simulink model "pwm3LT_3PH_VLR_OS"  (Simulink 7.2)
settings: Solver=ode3  SolverMode=SingleTasking  StartTime=0.0  StopTime=0.1  FixedStep=10e-6  MaxStep=1e-4  RelTol=1e-3

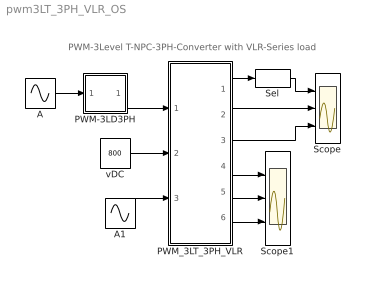
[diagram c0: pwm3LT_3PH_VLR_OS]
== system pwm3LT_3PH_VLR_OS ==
  note: PWM-3Level T-NPC-3PH-Converter with VLR-Series load
  A : Sin  Amplitude=.8  Frequency=2*pi*50  Phase="[0  -2*pi/3  -4*pi/3 ]"  SampleTime=0
  A1 : Sin  Amplitude=0  Frequency=2*pi*50  Phase="[0  -2*pi/3  -4*pi/3 ]"  SampleTime=0
  PWM-3LD3PH : Subsystem  mask(PWM-3LD3PH){FT=900, PHT=0, A=0.5, O1=0.5, O2=-0.5, DT=1e-6}
      mask prompts: FT "Frequency of Trian Sig."; PHT "Phase Angle of Trian. Sig."; A "Amplitude of Trian. Sig."; O1 "Offset of 1st Trian"; O2 "Offset of 2nd Trian."; DT "Dead Time"
      mask help: Pulse Width Modulation for 3 Phase 3 Level Neutral point clamped Converter
  PWM_3LT_3PH_VLR : Subsystem  mask(pwm_3LT_3PH_VLR_OS){RL=1, LL=1e-3}
      mask prompts: RL "Load Resistance"; LL "Load Inductance"
      mask help: Open Source 3-Level T-NPC PWM_3PH Converter with VLR load Input Vector u: u{0:11}= gating Signals u[12]/2= VDC1, VDC2 u{13:15}= EA,EB,EC Output Vector y: y{0:2}= Va,Vb,Vc, Output AC Voltages to middle point y{3:5}= Ia,Ib,Ic, Output AC Currents y[6]= Vab.V, Output Voltage y{7:9} = T1.I,D1.I,T1.V y{10:12}= T2.I,D2.I,T2.V y[13]= D5.I y[14]= D5.V y[15]= IDC1, Input DC Current y[16]= IDC2, Input DC Current Parameter Vector p: p[0]=RL p[1]=LL You can pause the simulation during running, change the Parameters you want and continue the Simulation
  Scope : Scope  NumInputPorts=3
  Scope1 : Scope  NumInputPorts=3
  Sel : Selector  InputPortWidth=3  IndexOptions=Index vector (dialog)  Indices=[1 ]  OutputSizes=1
  vDC : Constant  Value=800  OutDataType=sfix(16)  OutScaling=2^0
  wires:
  A/1 -> PWM-3LD3PH/1(In1)
  A1/1 -> PWM_3LT_3PH_VLR/3(E_ABC)
  vDC/1 -> PWM_3LT_3PH_VLR/2(vDC)
  PWM-3LD3PH/1(Out1) -> PWM_3LT_3PH_VLR/1(Sw)
  PWM_3LT_3PH_VLR/4("iT1, iD1,vT1") -> Scope1/1
  PWM_3LT_3PH_VLR/5("iT2, iD2,vT2") -> Scope1/2
  PWM_3LT_3PH_VLR/6(iDC1,iDC2) -> Scope1/3
  PWM_3LT_3PH_VLR/1(vABC) -> Sel/1
  PWM_3LT_3PH_VLR/2(iABC) -> Scope/2
  PWM_3LT_3PH_VLR/3(vAB) -> Scope/3
  Sel/1 -> Scope/1

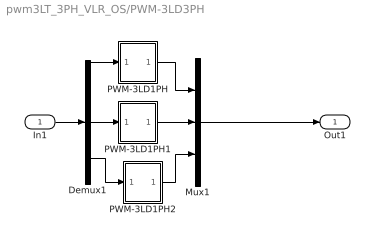
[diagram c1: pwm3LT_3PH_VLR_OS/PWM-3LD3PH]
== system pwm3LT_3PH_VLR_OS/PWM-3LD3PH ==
  In1 : Inport  OutDataType=sfix(16)  OutScaling=2^0
  Demux1 : Demux  Outputs=3
  Mux1 : Mux  Inputs=3
  PWM-3LD1PH : Subsystem  mask(PWM-3LD_1PH){FT=FT, PHT=PHT, A=A, O1=O1, O2=O2, DT=DT}
      mask prompts: FT "Frequency of Trian Sig."; PHT "Phase Angle of Trian. Sig."; A "Amplitude of Trian. Sig."; O1 "Offset of 1st Trian"; O2 "Offset of 2nd Trian."; DT "Dead Time"
      mask help: Pulse Width Modulation for 1 Leg of 3 Level Neutral point clamped Converter
  PWM-3LD1PH1 : Subsystem  mask(PWM-3LD_1PH){FT=FT, PHT=PHT, A=A, O1=O1, O2=O2, DT=DT}
      mask prompts: FT "Frequency of Trian Sig."; PHT "Phase Angle of Trian. Sig."; A "Amplitude of Trian. Sig."; O1 "Offset of 1st Trian"; O2 "Offset of 2nd Trian."; DT "Dead Time"
      mask help: Pulse Width Modulation for 1 Leg of 3 Level Neutral point clamped Converter
  PWM-3LD1PH2 : Subsystem  mask(PWM-3LD_1PH){FT=FT, PHT=PHT, A=A, O1=O1, O2=O2, DT=DT}
      mask prompts: FT "Frequency of Trian Sig."; PHT "Phase Angle of Trian. Sig."; A "Amplitude of Trian. Sig."; O1 "Offset of 1st Trian"; O2 "Offset of 2nd Trian."; DT "Dead Time"
      mask help: Pulse Width Modulation for 1 Leg of 3 Level Neutral point clamped Converter
  Out1 : Outport
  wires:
  In1/1 -> Demux1/1
  Demux1/3 -> PWM-3LD1PH2/1(In1)
  Demux1/2 -> PWM-3LD1PH1/1(In1)
  Demux1/1 -> PWM-3LD1PH/1(In1)
  Mux1/1 -> Out1/1
  PWM-3LD1PH2/1(Out1) -> Mux1/3
  PWM-3LD1PH1/1(Out1) -> Mux1/2
  PWM-3LD1PH/1(Out1) -> Mux1/1

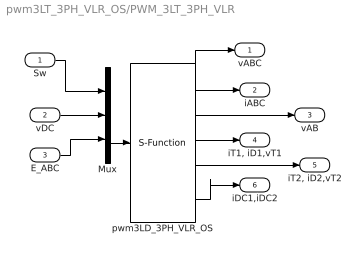
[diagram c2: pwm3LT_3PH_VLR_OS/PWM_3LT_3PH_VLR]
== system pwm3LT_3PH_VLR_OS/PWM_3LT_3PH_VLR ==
  Sw : Inport  OutDataType=sfix(16)  OutScaling=2^0
  vDC : Inport  Port=2  OutDataType=sfix(16)  OutScaling=2^0
  E_ABC : Inport  Port=3  OutDataType=sfix(16)  OutScaling=2^0
  Mux : Mux  Inputs="[12 1  3]"
  pwm3LD_3PH_VLR_OS : S-Function  FunctionName=s_pwm_3LT_3PH_VLR_OS  Parameters="[RL  LL]"  EnableBusSupport=off
  vABC : Outport  OutDataType=sfix(16)  OutScaling=2^0
  iABC : Outport  Port=2  OutDataType=sfix(16)  OutScaling=2^0
  vAB : Outport  Port=3  OutDataType=sfix(16)  OutScaling=2^0
  "iT1, iD1,vT1" : Outport  Port=4  OutDataType=sfix(16)  OutScaling=2^0
  "iT2, iD2,vT2" : Outport  Port=5  OutDataType=sfix(16)  OutScaling=2^0
  iDC1,iDC2 : Outport  Port=6  OutDataType=sfix(16)  OutScaling=2^0
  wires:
  Sw/1 -> Mux/1
  vDC/1 -> Mux/2
  Mux/1 -> pwm3LD_3PH_VLR_OS/1
  E_ABC/1 -> Mux/3
  pwm3LD_3PH_VLR_OS/1 -> vABC/1
  pwm3LD_3PH_VLR_OS/4 -> "iT1, iD1,vT1"/1
  pwm3LD_3PH_VLR_OS/2 -> iABC/1
  pwm3LD_3PH_VLR_OS/3 -> vAB/1
  pwm3LD_3PH_VLR_OS/5 -> "iT2, iD2,vT2"/1
  pwm3LD_3PH_VLR_OS/6 -> iDC1,iDC2/1

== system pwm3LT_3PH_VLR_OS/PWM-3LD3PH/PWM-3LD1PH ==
  In1 : Inport  OutDataType=sfix(16)  OutScaling=2^0
  Mux : Mux
  SS : Subsystem
  SS1 : Subsystem
  Out1 : Outport
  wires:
  In1/1 -> SS1/1(I1), SS/1(I1)
  SS1/1(O1) -> Mux/2
  SS/2(O2) -> Mux/3
  Mux/1 -> Out1/1
  SS/1(O1) -> Mux/1
  SS1/2(O2) -> Mux/4

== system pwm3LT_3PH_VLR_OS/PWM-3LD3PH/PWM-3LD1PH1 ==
  In1 : Inport  OutDataType=sfix(16)  OutScaling=2^0
  Mux : Mux
  SS : Subsystem
  SS1 : Subsystem
  Out1 : Outport
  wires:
  SS1/2(O2) -> Mux/4
  SS/1(O1) -> Mux/1
  Mux/1 -> Out1/1
  SS/2(O2) -> Mux/3
  SS1/1(O1) -> Mux/2
  In1/1 -> SS/1(I1), SS1/1(I1)

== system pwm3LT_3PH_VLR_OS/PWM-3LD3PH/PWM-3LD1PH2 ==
  In1 : Inport  OutDataType=sfix(16)  OutScaling=2^0
  Mux : Mux
  SS : Subsystem
  SS1 : Subsystem
  Out1 : Outport
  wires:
  In1/1 -> SS1/1(I1), SS/1(I1)
  SS1/1(O1) -> Mux/2
  SS/2(O2) -> Mux/3
  Mux/1 -> Out1/1
  SS/1(O1) -> Mux/1
  SS1/2(O2) -> Mux/4

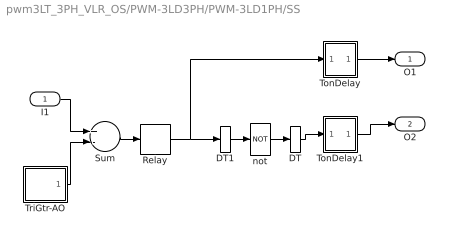
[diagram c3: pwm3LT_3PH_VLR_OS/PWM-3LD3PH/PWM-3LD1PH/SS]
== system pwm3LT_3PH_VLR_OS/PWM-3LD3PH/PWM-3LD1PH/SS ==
  I1 : Inport  OutDataType=sfix(16)  OutScaling=2^0
  DT : DataTypeConversion
  DT1 : DataTypeConversion
  Relay : Relay  OutDataType=sfix(16)  OutScaling=2^0
  Sum : Sum  Inputs=+-  OutDataType=sfix(16)  OutScaling=2^0
  TonDelay : Subsystem  mask(TonDelay){DT=DT}
      mask prompts: DT "Dead Time"
      mask help: Turn on dead time to protect against short circuit of the converter leg
  TonDelay1 : Subsystem  mask(TonDelay){DT=DT}
      mask prompts: DT "Dead Time"
      mask help: Turn on dead time to protect against short circuit of the converter leg
  TriGtr-AO : Subsystem  mask(TriGtr-AO){A=A, O=O1, T=1/FT, Td=PHT/FT/180}
      mask prompts: A "Amplitude"; O "Offset"; T "Period Time"; Td "Time Delay"
      mask help: Triangular Wave Generator with variable time delay, variable amplitude and offset
  not : Logic  Operator=NOT  Inputs=1
  O1 : Outport  InitialOutput=0
  O2 : Outport  Port=2  InitialOutput=0
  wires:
  TonDelay/1(s1d) -> O1/1
  Relay/1 -> TonDelay/1(s1), DT1/1
  TonDelay1/1(s1d) -> O2/1
  not/1 -> DT/1
  Sum/1 -> Relay/1
  TriGtr-AO/1(Out1) -> Sum/2
  I1/1 -> Sum/1
  DT/1 -> TonDelay1/1(s1)
  DT1/1 -> not/1

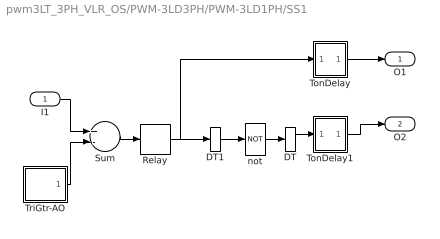
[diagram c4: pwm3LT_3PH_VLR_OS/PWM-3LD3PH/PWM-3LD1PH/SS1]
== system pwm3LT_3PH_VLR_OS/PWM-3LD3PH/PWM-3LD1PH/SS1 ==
  I1 : Inport  OutDataType=sfix(16)  OutScaling=2^0
  DT : DataTypeConversion
  DT1 : DataTypeConversion
  Relay : Relay  OutDataType=sfix(16)  OutScaling=2^0
  Sum : Sum  Inputs=+-  OutDataType=sfix(16)  OutScaling=2^0
  TonDelay : Subsystem  mask(TonDelay){DT=DT}
      mask prompts: DT "Dead Time"
      mask help: Turn on dead time to protect against short circuit of the converter leg
  TonDelay1 : Subsystem  mask(TonDelay){DT=DT}
      mask prompts: DT "Dead Time"
      mask help: Turn on dead time to protect against short circuit of the converter leg
  TriGtr-AO : Subsystem  mask(TriGtr-AO){A=A, O=O2, T=1/FT, Td=PHT/FT/180}
      mask prompts: A "Amplitude"; O "Offset"; T "Period Time"; Td "Time Delay"
      mask help: Triangular Wave Generator with variable time delay, variable amplitude and offset
  not : Logic  Operator=NOT  Inputs=1
  O1 : Outport  InitialOutput=0
  O2 : Outport  Port=2  InitialOutput=0
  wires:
  TonDelay/1(s1d) -> O1/1
  Relay/1 -> TonDelay/1(s1), DT1/1
  TonDelay1/1(s1d) -> O2/1
  not/1 -> DT/1
  Sum/1 -> Relay/1
  TriGtr-AO/1(Out1) -> Sum/2
  I1/1 -> Sum/1
  DT/1 -> TonDelay1/1(s1)
  DT1/1 -> not/1

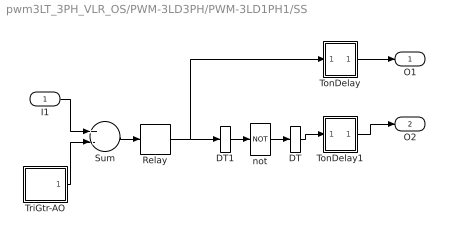
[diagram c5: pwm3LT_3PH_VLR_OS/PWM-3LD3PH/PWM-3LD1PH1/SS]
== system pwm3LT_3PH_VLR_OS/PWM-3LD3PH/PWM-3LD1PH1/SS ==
  I1 : Inport  OutDataType=sfix(16)  OutScaling=2^0
  DT : DataTypeConversion
  DT1 : DataTypeConversion
  Relay : Relay  OutDataType=sfix(16)  OutScaling=2^0
  Sum : Sum  Inputs=+-  OutDataType=sfix(16)  OutScaling=2^0
  TonDelay : Subsystem  mask(TonDelay){DT=DT}
      mask prompts: DT "Dead Time"
      mask help: Turn on dead time to protect against short circuit of the converter leg
  TonDelay1 : Subsystem  mask(TonDelay){DT=DT}
      mask prompts: DT "Dead Time"
      mask help: Turn on dead time to protect against short circuit of the converter leg
  TriGtr-AO : Subsystem  mask(TriGtr-AO){A=A, O=O1, T=1/FT, Td=PHT/FT/180}
      mask prompts: A "Amplitude"; O "Offset"; T "Period Time"; Td "Time Delay"
      mask help: Triangular Wave Generator with variable time delay, variable amplitude and offset
  not : Logic  Operator=NOT  Inputs=1
  O1 : Outport  InitialOutput=0
  O2 : Outport  Port=2  InitialOutput=0
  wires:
  DT1/1 -> not/1
  DT/1 -> TonDelay1/1(s1)
  I1/1 -> Sum/1
  TriGtr-AO/1(Out1) -> Sum/2
  Sum/1 -> Relay/1
  not/1 -> DT/1
  TonDelay1/1(s1d) -> O2/1
  Relay/1 -> DT1/1, TonDelay/1(s1)
  TonDelay/1(s1d) -> O1/1

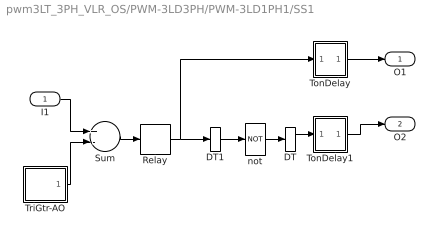
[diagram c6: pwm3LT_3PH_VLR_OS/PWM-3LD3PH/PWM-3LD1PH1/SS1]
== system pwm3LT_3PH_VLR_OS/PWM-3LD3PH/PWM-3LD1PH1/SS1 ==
  I1 : Inport  OutDataType=sfix(16)  OutScaling=2^0
  DT : DataTypeConversion
  DT1 : DataTypeConversion
  Relay : Relay  OutDataType=sfix(16)  OutScaling=2^0
  Sum : Sum  Inputs=+-  OutDataType=sfix(16)  OutScaling=2^0
  TonDelay : Subsystem  mask(TonDelay){DT=DT}
      mask prompts: DT "Dead Time"
      mask help: Turn on dead time to protect against short circuit of the converter leg
  TonDelay1 : Subsystem  mask(TonDelay){DT=DT}
      mask prompts: DT "Dead Time"
      mask help: Turn on dead time to protect against short circuit of the converter leg
  TriGtr-AO : Subsystem  mask(TriGtr-AO){A=A, O=O2, T=1/FT, Td=PHT/FT/180}
      mask prompts: A "Amplitude"; O "Offset"; T "Period Time"; Td "Time Delay"
      mask help: Triangular Wave Generator with variable time delay, variable amplitude and offset
  not : Logic  Operator=NOT  Inputs=1
  O1 : Outport  InitialOutput=0
  O2 : Outport  Port=2  InitialOutput=0
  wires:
  DT1/1 -> not/1
  DT/1 -> TonDelay1/1(s1)
  I1/1 -> Sum/1
  TriGtr-AO/1(Out1) -> Sum/2
  Sum/1 -> Relay/1
  not/1 -> DT/1
  TonDelay1/1(s1d) -> O2/1
  Relay/1 -> DT1/1, TonDelay/1(s1)
  TonDelay/1(s1d) -> O1/1

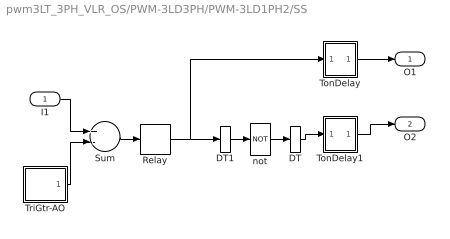
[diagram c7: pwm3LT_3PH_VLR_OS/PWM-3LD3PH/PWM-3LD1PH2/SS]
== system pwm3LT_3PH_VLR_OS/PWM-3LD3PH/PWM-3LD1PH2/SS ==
  I1 : Inport  OutDataType=sfix(16)  OutScaling=2^0
  DT : DataTypeConversion
  DT1 : DataTypeConversion
  Relay : Relay  OutDataType=sfix(16)  OutScaling=2^0
  Sum : Sum  Inputs=+-  OutDataType=sfix(16)  OutScaling=2^0
  TonDelay : Subsystem  mask(TonDelay){DT=DT}
      mask prompts: DT "Dead Time"
      mask help: Turn on dead time to protect against short circuit of the converter leg
  TonDelay1 : Subsystem  mask(TonDelay){DT=DT}
      mask prompts: DT "Dead Time"
      mask help: Turn on dead time to protect against short circuit of the converter leg
  TriGtr-AO : Subsystem  mask(TriGtr-AO){A=A, O=O1, T=1/FT, Td=PHT/FT/180}
      mask prompts: A "Amplitude"; O "Offset"; T "Period Time"; Td "Time Delay"
      mask help: Triangular Wave Generator with variable time delay, variable amplitude and offset
  not : Logic  Operator=NOT  Inputs=1
  O1 : Outport  InitialOutput=0
  O2 : Outport  Port=2  InitialOutput=0
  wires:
  TonDelay/1(s1d) -> O1/1
  Relay/1 -> TonDelay/1(s1), DT1/1
  TonDelay1/1(s1d) -> O2/1
  not/1 -> DT/1
  Sum/1 -> Relay/1
  TriGtr-AO/1(Out1) -> Sum/2
  I1/1 -> Sum/1
  DT/1 -> TonDelay1/1(s1)
  DT1/1 -> not/1

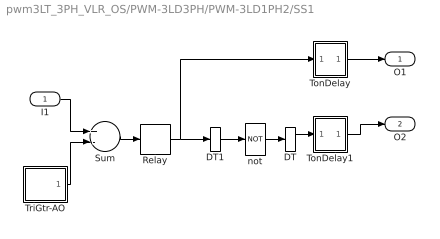
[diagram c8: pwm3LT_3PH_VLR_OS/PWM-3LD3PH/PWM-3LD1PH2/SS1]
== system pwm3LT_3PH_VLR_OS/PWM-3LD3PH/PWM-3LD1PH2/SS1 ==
  I1 : Inport  OutDataType=sfix(16)  OutScaling=2^0
  DT : DataTypeConversion
  DT1 : DataTypeConversion
  Relay : Relay  OutDataType=sfix(16)  OutScaling=2^0
  Sum : Sum  Inputs=+-  OutDataType=sfix(16)  OutScaling=2^0
  TonDelay : Subsystem  mask(TonDelay){DT=DT}
      mask prompts: DT "Dead Time"
      mask help: Turn on dead time to protect against short circuit of the converter leg
  TonDelay1 : Subsystem  mask(TonDelay){DT=DT}
      mask prompts: DT "Dead Time"
      mask help: Turn on dead time to protect against short circuit of the converter leg
  TriGtr-AO : Subsystem  mask(TriGtr-AO){A=A, O=O2, T=1/FT, Td=PHT/FT/180}
      mask prompts: A "Amplitude"; O "Offset"; T "Period Time"; Td "Time Delay"
      mask help: Triangular Wave Generator with variable time delay, variable amplitude and offset
  not : Logic  Operator=NOT  Inputs=1
  O1 : Outport  InitialOutput=0
  O2 : Outport  Port=2  InitialOutput=0
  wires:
  TonDelay/1(s1d) -> O1/1
  Relay/1 -> TonDelay/1(s1), DT1/1
  TonDelay1/1(s1d) -> O2/1
  not/1 -> DT/1
  Sum/1 -> Relay/1
  TriGtr-AO/1(Out1) -> Sum/2
  I1/1 -> Sum/1
  DT/1 -> TonDelay1/1(s1)
  DT1/1 -> not/1

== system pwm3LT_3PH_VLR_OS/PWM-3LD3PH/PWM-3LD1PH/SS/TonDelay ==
  s1 : Inport  Orientation=down  OutDataType=sfix(16)  OutScaling=2^0
  Int : Integrator  ExternalReset=falling
  Rel1 : Relay  OnSwitchValue=DT  OutDataType=sfix(16)  OutScaling=2^0
  s1d : Outport  InitialOutput=0
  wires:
  Rel1/1 -> s1d/1
  s1/1 -> Int/1, Int/2
  Int/1 -> Rel1/1

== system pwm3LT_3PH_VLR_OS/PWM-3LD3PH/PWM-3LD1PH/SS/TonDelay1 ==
  s1 : Inport  Orientation=down  OutDataType=sfix(16)  OutScaling=2^0
  Int : Integrator  ExternalReset=falling
  Rel1 : Relay  OnSwitchValue=DT  OutDataType=sfix(16)  OutScaling=2^0
  s1d : Outport  InitialOutput=0
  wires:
  Rel1/1 -> s1d/1
  s1/1 -> Int/1, Int/2
  Int/1 -> Rel1/1

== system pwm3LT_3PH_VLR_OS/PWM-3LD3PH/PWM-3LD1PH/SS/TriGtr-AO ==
  Ampl. : Gain  Gain=A  ParameterDataType=sfix(16)  ParameterScaling=2^0  OutDataType=sfix(16)  OutScaling=2^0
  Offset : Constant  Value=O  OutDataType=sfix(16)  OutScaling=2^0
  Sum : Sum  OutDataType=sfix(16)  OutScaling=2^0
  TriGtr1 : Subsystem  mask(TriGtr){T=T, Td=Td}
      mask prompts: T "Period Time"; Td "Time Delay"
      mask help: Triangular Wave Generator with variable time delay
  Out1 : Outport
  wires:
  Sum/1 -> Out1/1
  Ampl./1 -> Sum/1
  TriGtr1/1(O) -> Ampl./1
  Offset/1 -> Sum/2

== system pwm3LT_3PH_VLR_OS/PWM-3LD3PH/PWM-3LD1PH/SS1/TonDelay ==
  s1 : Inport  Orientation=down  OutDataType=sfix(16)  OutScaling=2^0
  Int : Integrator  ExternalReset=falling
  Rel1 : Relay  OnSwitchValue=DT  OutDataType=sfix(16)  OutScaling=2^0
  s1d : Outport  InitialOutput=0
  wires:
  Rel1/1 -> s1d/1
  s1/1 -> Int/1, Int/2
  Int/1 -> Rel1/1

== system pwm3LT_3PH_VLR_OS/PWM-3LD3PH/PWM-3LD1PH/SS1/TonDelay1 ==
  s1 : Inport  Orientation=down  OutDataType=sfix(16)  OutScaling=2^0
  Int : Integrator  ExternalReset=falling
  Rel1 : Relay  OnSwitchValue=DT  OutDataType=sfix(16)  OutScaling=2^0
  s1d : Outport  InitialOutput=0
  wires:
  Rel1/1 -> s1d/1
  s1/1 -> Int/1, Int/2
  Int/1 -> Rel1/1

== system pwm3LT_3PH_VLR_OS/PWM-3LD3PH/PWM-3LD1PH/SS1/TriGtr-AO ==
  Ampl. : Gain  Gain=A  ParameterDataType=sfix(16)  ParameterScaling=2^0  OutDataType=sfix(16)  OutScaling=2^0
  Offset : Constant  Value=O  OutDataType=sfix(16)  OutScaling=2^0
  Sum : Sum  OutDataType=sfix(16)  OutScaling=2^0
  TriGtr1 : Subsystem  mask(TriGtr){T=T, Td=Td}
      mask prompts: T "Period Time"; Td "Time Delay"
      mask help: Triangular Wave Generator with variable time delay
  Out1 : Outport
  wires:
  Offset/1 -> Sum/2
  TriGtr1/1(O) -> Ampl./1
  Ampl./1 -> Sum/1
  Sum/1 -> Out1/1

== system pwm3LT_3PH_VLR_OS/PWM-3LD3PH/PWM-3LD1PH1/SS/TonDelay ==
  s1 : Inport  Orientation=down  OutDataType=sfix(16)  OutScaling=2^0
  Int : Integrator  ExternalReset=falling
  Rel1 : Relay  OnSwitchValue=DT  OutDataType=sfix(16)  OutScaling=2^0
  s1d : Outport  InitialOutput=0
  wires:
  Int/1 -> Rel1/1
  s1/1 -> Int/2, Int/1
  Rel1/1 -> s1d/1

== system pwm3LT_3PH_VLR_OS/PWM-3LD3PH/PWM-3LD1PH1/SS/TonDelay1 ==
  s1 : Inport  Orientation=down  OutDataType=sfix(16)  OutScaling=2^0
  Int : Integrator  ExternalReset=falling
  Rel1 : Relay  OnSwitchValue=DT  OutDataType=sfix(16)  OutScaling=2^0
  s1d : Outport  InitialOutput=0
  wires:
  Int/1 -> Rel1/1
  s1/1 -> Int/2, Int/1
  Rel1/1 -> s1d/1

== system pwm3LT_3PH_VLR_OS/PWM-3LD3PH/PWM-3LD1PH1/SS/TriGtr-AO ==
  Ampl. : Gain  Gain=A  ParameterDataType=sfix(16)  ParameterScaling=2^0  OutDataType=sfix(16)  OutScaling=2^0
  Offset : Constant  Value=O  OutDataType=sfix(16)  OutScaling=2^0
  Sum : Sum  OutDataType=sfix(16)  OutScaling=2^0
  TriGtr1 : Subsystem  mask(TriGtr){T=T, Td=Td}
      mask prompts: T "Period Time"; Td "Time Delay"
      mask help: Triangular Wave Generator with variable time delay
  Out1 : Outport
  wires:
  Offset/1 -> Sum/2
  TriGtr1/1(O) -> Ampl./1
  Ampl./1 -> Sum/1
  Sum/1 -> Out1/1

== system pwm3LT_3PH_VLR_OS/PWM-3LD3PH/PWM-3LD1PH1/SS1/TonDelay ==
  s1 : Inport  Orientation=down  OutDataType=sfix(16)  OutScaling=2^0
  Int : Integrator  ExternalReset=falling
  Rel1 : Relay  OnSwitchValue=DT  OutDataType=sfix(16)  OutScaling=2^0
  s1d : Outport  InitialOutput=0
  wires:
  Int/1 -> Rel1/1
  s1/1 -> Int/2, Int/1
  Rel1/1 -> s1d/1

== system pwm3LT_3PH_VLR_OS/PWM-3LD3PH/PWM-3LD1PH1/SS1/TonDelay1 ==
  s1 : Inport  Orientation=down  OutDataType=sfix(16)  OutScaling=2^0
  Int : Integrator  ExternalReset=falling
  Rel1 : Relay  OnSwitchValue=DT  OutDataType=sfix(16)  OutScaling=2^0
  s1d : Outport  InitialOutput=0
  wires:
  Int/1 -> Rel1/1
  s1/1 -> Int/2, Int/1
  Rel1/1 -> s1d/1

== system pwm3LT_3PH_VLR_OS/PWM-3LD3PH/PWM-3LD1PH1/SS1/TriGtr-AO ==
  Ampl. : Gain  Gain=A  ParameterDataType=sfix(16)  ParameterScaling=2^0  OutDataType=sfix(16)  OutScaling=2^0
  Offset : Constant  Value=O  OutDataType=sfix(16)  OutScaling=2^0
  Sum : Sum  OutDataType=sfix(16)  OutScaling=2^0
  TriGtr1 : Subsystem  mask(TriGtr){T=T, Td=Td}
      mask prompts: T "Period Time"; Td "Time Delay"
      mask help: Triangular Wave Generator with variable time delay
  Out1 : Outport
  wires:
  Sum/1 -> Out1/1
  Ampl./1 -> Sum/1
  TriGtr1/1(O) -> Ampl./1
  Offset/1 -> Sum/2

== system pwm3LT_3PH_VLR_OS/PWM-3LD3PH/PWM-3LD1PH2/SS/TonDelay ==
  s1 : Inport  Orientation=down  OutDataType=sfix(16)  OutScaling=2^0
  Int : Integrator  ExternalReset=falling
  Rel1 : Relay  OnSwitchValue=DT  OutDataType=sfix(16)  OutScaling=2^0
  s1d : Outport  InitialOutput=0
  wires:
  Rel1/1 -> s1d/1
  s1/1 -> Int/1, Int/2
  Int/1 -> Rel1/1

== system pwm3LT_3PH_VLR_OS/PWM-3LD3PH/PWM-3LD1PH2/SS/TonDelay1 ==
  s1 : Inport  Orientation=down  OutDataType=sfix(16)  OutScaling=2^0
  Int : Integrator  ExternalReset=falling
  Rel1 : Relay  OnSwitchValue=DT  OutDataType=sfix(16)  OutScaling=2^0
  s1d : Outport  InitialOutput=0
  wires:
  Rel1/1 -> s1d/1
  s1/1 -> Int/1, Int/2
  Int/1 -> Rel1/1

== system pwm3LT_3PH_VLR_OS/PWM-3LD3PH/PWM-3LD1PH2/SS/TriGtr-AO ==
  Ampl. : Gain  Gain=A  ParameterDataType=sfix(16)  ParameterScaling=2^0  OutDataType=sfix(16)  OutScaling=2^0
  Offset : Constant  Value=O  OutDataType=sfix(16)  OutScaling=2^0
  Sum : Sum  OutDataType=sfix(16)  OutScaling=2^0
  TriGtr1 : Subsystem  mask(TriGtr){T=T, Td=Td}
      mask prompts: T "Period Time"; Td "Time Delay"
      mask help: Triangular Wave Generator with variable time delay
  Out1 : Outport
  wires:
  Sum/1 -> Out1/1
  Ampl./1 -> Sum/1
  TriGtr1/1(O) -> Ampl./1
  Offset/1 -> Sum/2

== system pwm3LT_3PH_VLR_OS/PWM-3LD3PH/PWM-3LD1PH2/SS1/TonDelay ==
  s1 : Inport  Orientation=down  OutDataType=sfix(16)  OutScaling=2^0
  Int : Integrator  ExternalReset=falling
  Rel1 : Relay  OnSwitchValue=DT  OutDataType=sfix(16)  OutScaling=2^0
  s1d : Outport  InitialOutput=0
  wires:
  Rel1/1 -> s1d/1
  s1/1 -> Int/1, Int/2
  Int/1 -> Rel1/1

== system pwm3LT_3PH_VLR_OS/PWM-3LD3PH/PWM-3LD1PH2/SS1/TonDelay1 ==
  s1 : Inport  Orientation=down  OutDataType=sfix(16)  OutScaling=2^0
  Int : Integrator  ExternalReset=falling
  Rel1 : Relay  OnSwitchValue=DT  OutDataType=sfix(16)  OutScaling=2^0
  s1d : Outport  InitialOutput=0
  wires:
  Rel1/1 -> s1d/1
  s1/1 -> Int/1, Int/2
  Int/1 -> Rel1/1

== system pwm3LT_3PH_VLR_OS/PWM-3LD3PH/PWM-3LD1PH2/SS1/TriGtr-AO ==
  Ampl. : Gain  Gain=A  ParameterDataType=sfix(16)  ParameterScaling=2^0  OutDataType=sfix(16)  OutScaling=2^0
  Offset : Constant  Value=O  OutDataType=sfix(16)  OutScaling=2^0
  Sum : Sum  OutDataType=sfix(16)  OutScaling=2^0
  TriGtr1 : Subsystem  mask(TriGtr){T=T, Td=Td}
      mask prompts: T "Period Time"; Td "Time Delay"
      mask help: Triangular Wave Generator with variable time delay
  Out1 : Outport
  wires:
  Offset/1 -> Sum/2
  TriGtr1/1(O) -> Ampl./1
  Ampl./1 -> Sum/1
  Sum/1 -> Out1/1

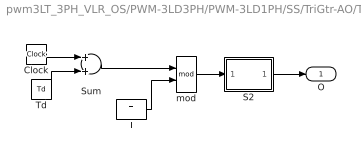
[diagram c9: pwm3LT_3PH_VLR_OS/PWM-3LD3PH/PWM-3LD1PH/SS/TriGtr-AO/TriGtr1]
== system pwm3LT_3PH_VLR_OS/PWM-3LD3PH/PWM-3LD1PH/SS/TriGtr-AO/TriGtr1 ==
  Clock : Clock
  S2 : Subsystem
  Sum : Sum  OutDataType=sfix(16)  OutScaling=2^0
  T : Constant  Value=T  OutDataType=sfix(16)  OutScaling=2^0
  Td : Constant  Value=Td  OutDataType=sfix(16)  OutScaling=2^0
  mod : Math  Operator=mod
  O : Outport  InitialOutput=0
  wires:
  Td/1 -> Sum/2
  Sum/1 -> mod/1
  T/1 -> mod/2
  Clock/1 -> Sum/1
  S2/1(O1) -> O/1
  mod/1 -> S2/1(I1)

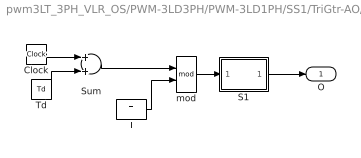
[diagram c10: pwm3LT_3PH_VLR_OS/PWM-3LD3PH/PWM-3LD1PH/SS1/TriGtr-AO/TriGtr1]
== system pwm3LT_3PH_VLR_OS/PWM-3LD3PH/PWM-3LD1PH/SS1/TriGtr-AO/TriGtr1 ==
  Clock : Clock
  S1 : Subsystem
  Sum : Sum
  T : Constant  Value=T
  Td : Constant  Value=Td
  mod : Math  Operator=mod
  O : Outport  InitialOutput=0
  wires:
  Td/1 -> Sum/2
  Sum/1 -> mod/1
  T/1 -> mod/2
  Clock/1 -> Sum/1
  S1/1(O1) -> O/1
  mod/1 -> S1/1(I1)

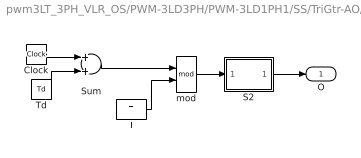
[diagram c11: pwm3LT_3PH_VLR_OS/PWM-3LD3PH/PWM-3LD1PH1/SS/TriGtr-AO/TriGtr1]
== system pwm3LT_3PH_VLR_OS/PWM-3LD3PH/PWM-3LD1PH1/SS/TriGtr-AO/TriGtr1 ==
  Clock : Clock
  S2 : Subsystem
  Sum : Sum  OutDataType=sfix(16)  OutScaling=2^0
  T : Constant  Value=T  OutDataType=sfix(16)  OutScaling=2^0
  Td : Constant  Value=Td  OutDataType=sfix(16)  OutScaling=2^0
  mod : Math  Operator=mod
  O : Outport  InitialOutput=0
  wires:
  mod/1 -> S2/1(I1)
  S2/1(O1) -> O/1
  Clock/1 -> Sum/1
  T/1 -> mod/2
  Sum/1 -> mod/1
  Td/1 -> Sum/2

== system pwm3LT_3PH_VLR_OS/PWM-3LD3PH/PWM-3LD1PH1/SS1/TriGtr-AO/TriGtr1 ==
  Clock : Clock
  S1 : Subsystem
  Sum : Sum
  T : Constant  Value=T
  Td : Constant  Value=Td
  mod : Math  Operator=mod
  O : Outport  InitialOutput=0
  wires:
  mod/1 -> S1/1(I1)
  S1/1(O1) -> O/1
  Clock/1 -> Sum/1
  T/1 -> mod/2
  Sum/1 -> mod/1
  Td/1 -> Sum/2

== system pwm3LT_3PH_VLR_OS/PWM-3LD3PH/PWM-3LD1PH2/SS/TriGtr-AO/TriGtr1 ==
  Clock : Clock
  S2 : Subsystem
  Sum : Sum  OutDataType=sfix(16)  OutScaling=2^0
  T : Constant  Value=T  OutDataType=sfix(16)  OutScaling=2^0
  Td : Constant  Value=Td  OutDataType=sfix(16)  OutScaling=2^0
  mod : Math  Operator=mod
  O : Outport  InitialOutput=0
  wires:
  Td/1 -> Sum/2
  Sum/1 -> mod/1
  T/1 -> mod/2
  Clock/1 -> Sum/1
  S2/1(O1) -> O/1
  mod/1 -> S2/1(I1)

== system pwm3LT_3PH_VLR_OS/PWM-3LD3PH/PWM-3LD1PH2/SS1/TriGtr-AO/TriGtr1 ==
  Clock : Clock
  S1 : Subsystem
  Sum : Sum
  T : Constant  Value=T
  Td : Constant  Value=Td
  mod : Math  Operator=mod
  O : Outport  InitialOutput=0
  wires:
  Td/1 -> Sum/2
  Sum/1 -> mod/1
  T/1 -> mod/2
  Clock/1 -> Sum/1
  S1/1(O1) -> O/1
  mod/1 -> S1/1(I1)

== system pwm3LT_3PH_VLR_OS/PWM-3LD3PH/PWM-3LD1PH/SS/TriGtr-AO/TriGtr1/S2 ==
  I1 : Inport
  Fcn : Fcn  Expr="(u* (u <=T/4) * 4/T)   +  (  (u > T/4) && ( u <=3*T/4) )* ( 1 - (u-T/4) *4/T )   +  ( (u > 3*T/4)&& (u<=T)) * ( ((u -3*T/4)* 4/T )-1 )"
  O1 : Outport
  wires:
  Fcn/1 -> O1/1
  I1/1 -> Fcn/1

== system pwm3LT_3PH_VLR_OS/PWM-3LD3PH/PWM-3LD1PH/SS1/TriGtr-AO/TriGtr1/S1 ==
  I1 : Inport
  Fcn : Fcn  Expr="(u* (u <=T/4) * 4/T)   +  (  (u > T/4) && ( u <=3*T/4) )* ( 1 - (u-T/4) *4/T )   +  ( (u > 3*T/4)&& (u<=T)) * ( ((u -3*T/4)* 4/T )-1 )"
  O1 : Outport
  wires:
  I1/1 -> Fcn/1
  Fcn/1 -> O1/1

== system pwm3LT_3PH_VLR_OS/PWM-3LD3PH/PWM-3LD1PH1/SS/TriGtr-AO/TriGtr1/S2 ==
  I1 : Inport
  Fcn : Fcn  Expr="(u* (u <=T/4) * 4/T)   +  (  (u > T/4) && ( u <=3*T/4) )* ( 1 - (u-T/4) *4/T )   +  ( (u > 3*T/4)&& (u<=T)) * ( ((u -3*T/4)* 4/T )-1 )"
  O1 : Outport
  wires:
  I1/1 -> Fcn/1
  Fcn/1 -> O1/1

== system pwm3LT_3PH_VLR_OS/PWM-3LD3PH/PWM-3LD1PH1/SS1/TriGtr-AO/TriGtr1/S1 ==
  I1 : Inport
  Fcn : Fcn  Expr="(u* (u <=T/4) * 4/T)   +  (  (u > T/4) && ( u <=3*T/4) )* ( 1 - (u-T/4) *4/T )   +  ( (u > 3*T/4)&& (u<=T)) * ( ((u -3*T/4)* 4/T )-1 )"
  O1 : Outport
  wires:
  Fcn/1 -> O1/1
  I1/1 -> Fcn/1

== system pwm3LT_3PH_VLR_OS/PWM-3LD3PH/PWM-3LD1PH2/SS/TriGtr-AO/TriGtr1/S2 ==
  I1 : Inport
  Fcn : Fcn  Expr="(u* (u <=T/4) * 4/T)   +  (  (u > T/4) && ( u <=3*T/4) )* ( 1 - (u-T/4) *4/T )   +  ( (u > 3*T/4)&& (u<=T)) * ( ((u -3*T/4)* 4/T )-1 )"
  O1 : Outport
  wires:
  Fcn/1 -> O1/1
  I1/1 -> Fcn/1

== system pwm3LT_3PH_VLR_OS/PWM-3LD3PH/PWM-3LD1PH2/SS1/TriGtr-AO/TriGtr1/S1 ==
  I1 : Inport
  Fcn : Fcn  Expr="(u* (u <=T/4) * 4/T)   +  (  (u > T/4) && ( u <=3*T/4) )* ( 1 - (u-T/4) *4/T )   +  ( (u > 3*T/4)&& (u<=T)) * ( ((u -3*T/4)* 4/T )-1 )"
  O1 : Outport
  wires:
  I1/1 -> Fcn/1
  Fcn/1 -> O1/1
